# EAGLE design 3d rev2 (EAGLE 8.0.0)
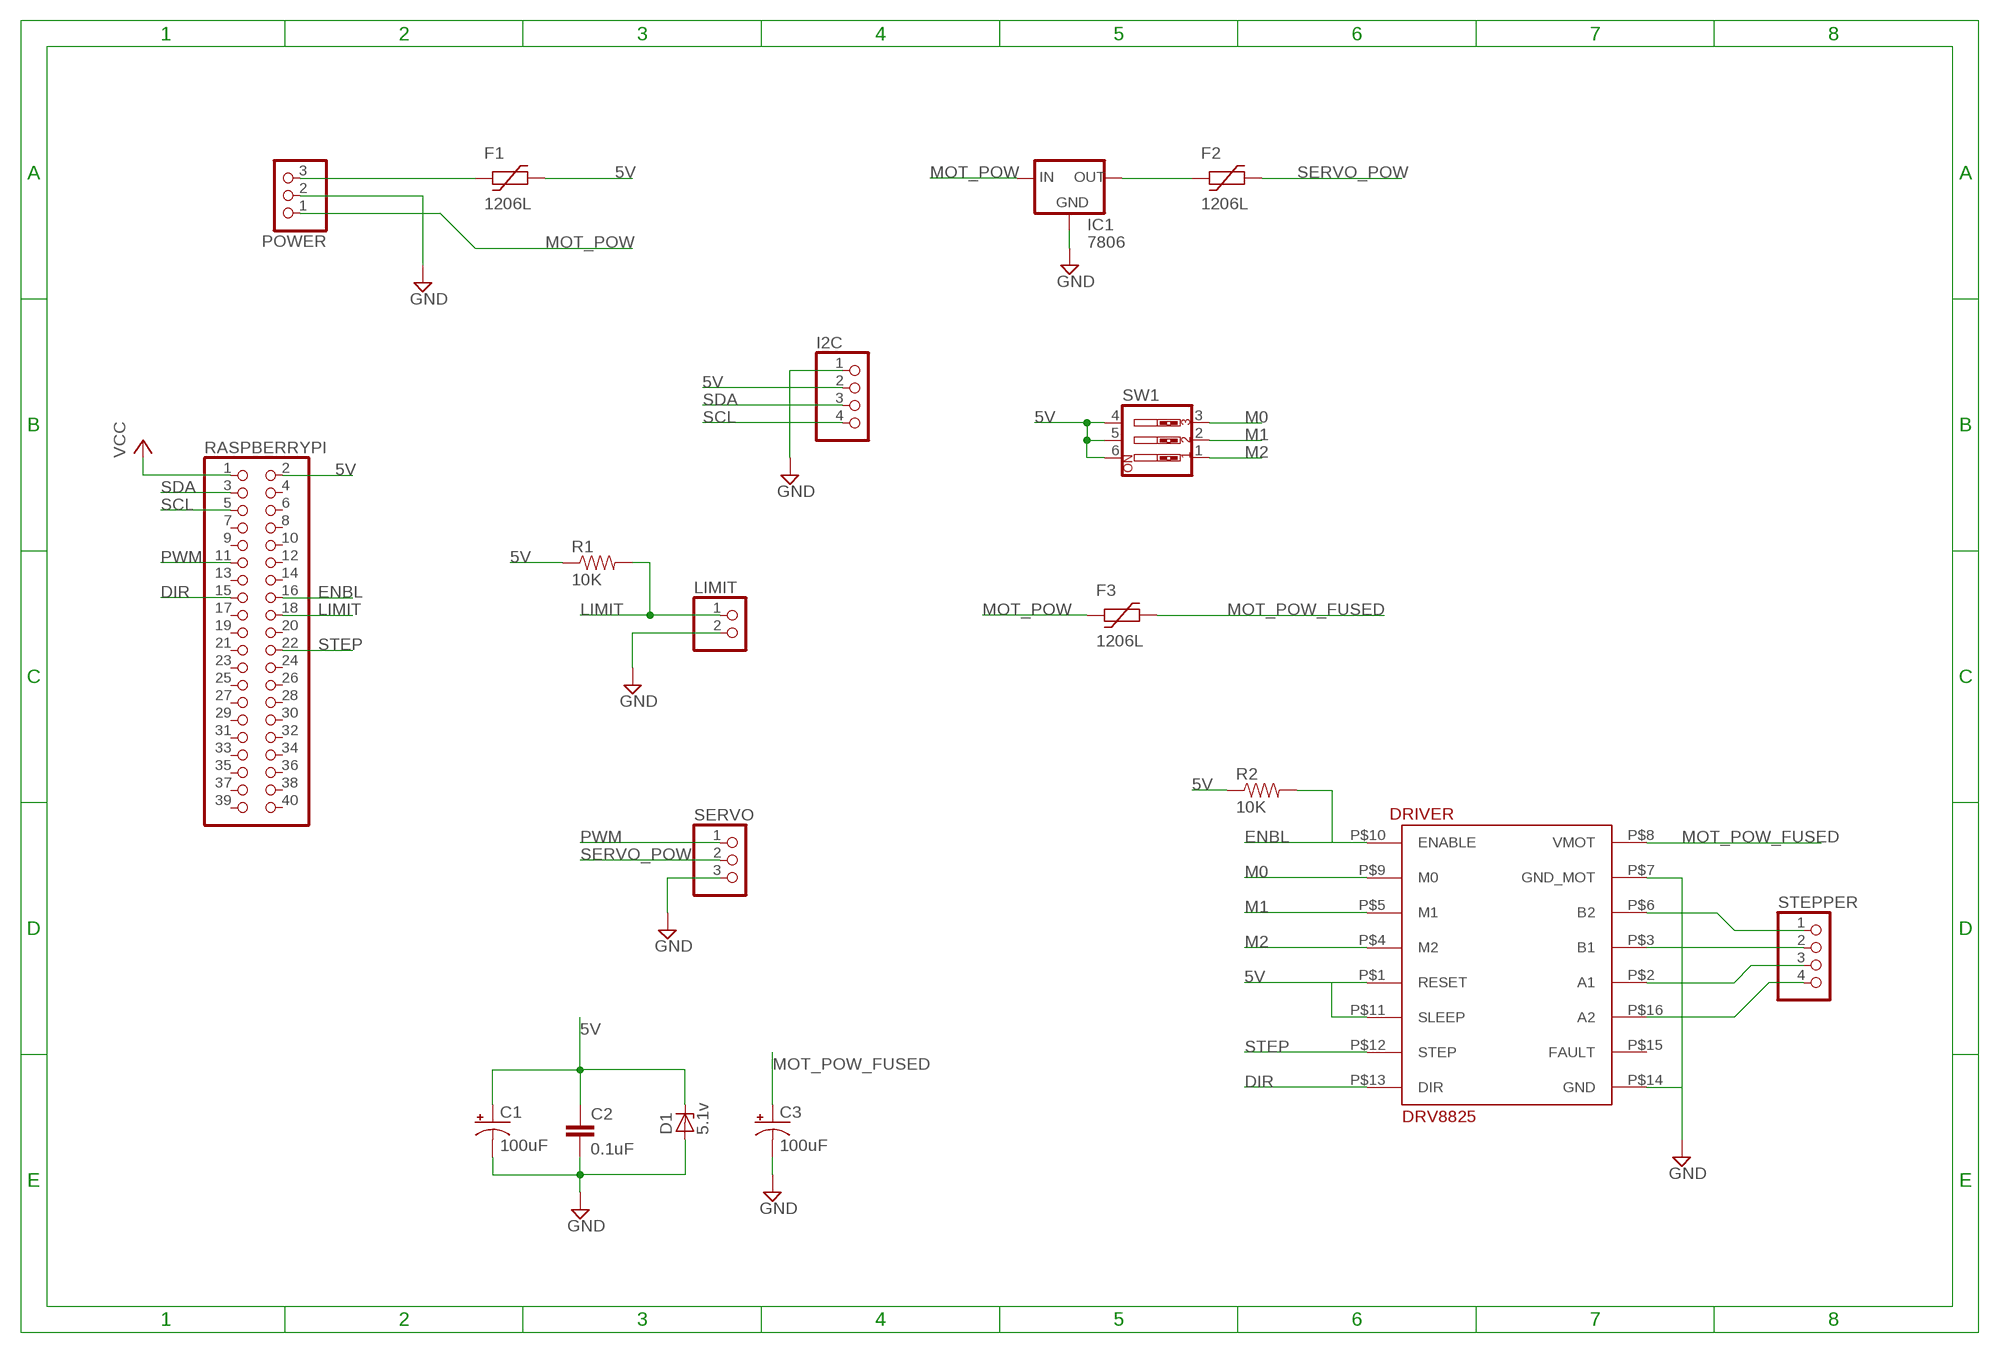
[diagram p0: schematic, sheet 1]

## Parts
C1  100uF  100UF-63V-20%(ELECT)  [NIC_10X10.5_CAP]
C2  0.1uF  0.1UF-25V-5%(0603)  [0603-CAP]
C3  100uF  100UF-63V-20%(ELECT)  [NIC_10X10.5_CAP]
D1  5.1v  ZENER-DIODESOD80C  [SOD80C]
DRIVER  DRV8825  [DRV8825]
F1  1206L  [1206L]
F2  1206L  [1206L]
F3  1206L  [1206L]
I2C  PINHD-1X4  [1X04]
IC1  7806  78LXX  [78LXX]
LIMIT  PINHD-1X2  [1X02]
POWER  PINHD-1X3  [1X03]
R1  10K  RESISTOR1206  [1206]
R2  10K  RESISTOR1206  [1206]
RASPBERRYPI  PINHD-2X20  [2X20]
SERVO  PINHD-1X3  [1X03]
STEPPER  PINHD-1X4  [1X04]
SW1  SW_DIP-3  [EDG-03]

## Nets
5V: C1.+ C2.1 D1.C DRIVER.P$1(RESET) DRIVER.P$11(SLEEP) F1.P$2 I2C.2 R1.1 R2.1 RASPBERRYPI.2 SW1.4 SW1.5 SW1.6
DIR: DRIVER.P$13(DIR) RASPBERRYPI.15
ENBL: DRIVER.P$10(ENABLE) R2.2 RASPBERRYPI.16
GND: C1.- C2.2 C3.- D1.A DRIVER.P$7(GND_MOT) DRIVER.P$14(GND) I2C.1 IC1.GND LIMIT.2 POWER.2 SERVO.3
LIMIT: LIMIT.1 R1.2 RASPBERRYPI.18
M0: DRIVER.P$9(M0) SW1.3
M1: DRIVER.P$5(M1) SW1.2
M2: DRIVER.P$4(M2) SW1.1
MOT_POW: F3.P$1 IC1.IN POWER.1
MOT_POW_FUSED: C3.+ DRIVER.P$8(VMOT) F3.P$2
N$1: DRIVER.P$6(B2) STEPPER.1
N$2: DRIVER.P$3(B1) STEPPER.2
N$3: DRIVER.P$2(A1) STEPPER.3
N$4: DRIVER.P$16(A2) STEPPER.4
N$7: F1.P$1 POWER.3
N$11: F2.P$1 IC1.OUT
PWM: RASPBERRYPI.11 SERVO.1
SCL: I2C.4 RASPBERRYPI.5
SDA: I2C.3 RASPBERRYPI.3
SERVO_POW: F2.P$2 SERVO.2
STEP: DRIVER.P$12(STEP) RASPBERRYPI.22
VCC: RASPBERRYPI.1
Unconnected: DRIVER.P$15(FAULT) RASPBERRYPI.4 RASPBERRYPI.6 RASPBERRYPI.7 RASPBERRYPI.8 RASPBERRYPI.9 RASPBERRYPI.10 RASPBERRYPI.12 RASPBERRYPI.13 RASPBERRYPI.14 RASPBERRYPI.17 RASPBERRYPI.19 RASPBERRYPI.20 RASPBERRYPI.21 RASPBERRYPI.23 RASPBERRYPI.24 RASPBERRYPI.25 RASPBERRYPI.26 RASPBERRYPI.27 RASPBERRYPI.28 RASPBERRYPI.29 RASPBERRYPI.30 RASPBERRYPI.31 RASPBERRYPI.32 RASPBERRYPI.33 RASPBERRYPI.34 RASPBERRYPI.35 RASPBERRYPI.36 RASPBERRYPI.37 RASPBERRYPI.38 RASPBERRYPI.39 RASPBERRYPI.40

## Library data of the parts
C1 C3 = SparkFun-Capacitors:100UF-63V-20%(ELECT): CAP-08362; PROD_ID: CAP-08362
C2 = SparkFun-Capacitors:0.1UF-25V-5%(0603): CAP-08604; PROD_ID: CAP-08604
D1 = diode:ZENER-DIODE: Z-Diode
DRIVER = drv8825 rev2:DRV8825
F1-F3 = ptc-littlefuse:1206L
I2C STEPPER = pinhead:PINHD-1X4: PIN HEADER
IC1 = v-reg:78LXX: VOLTAGE REGULATOR
LIMIT = pinhead:PINHD-1X2: PIN HEADER
POWER SERVO = pinhead:PINHD-1X3: PIN HEADER
R1 R2 = SparkFun-Resistors:RESISTOR: Resistor
RASPBERRYPI = pinhead:PINHD-2X20: PIN HEADER
SW1 = special:SW_DIP-3: DIP SWITCH

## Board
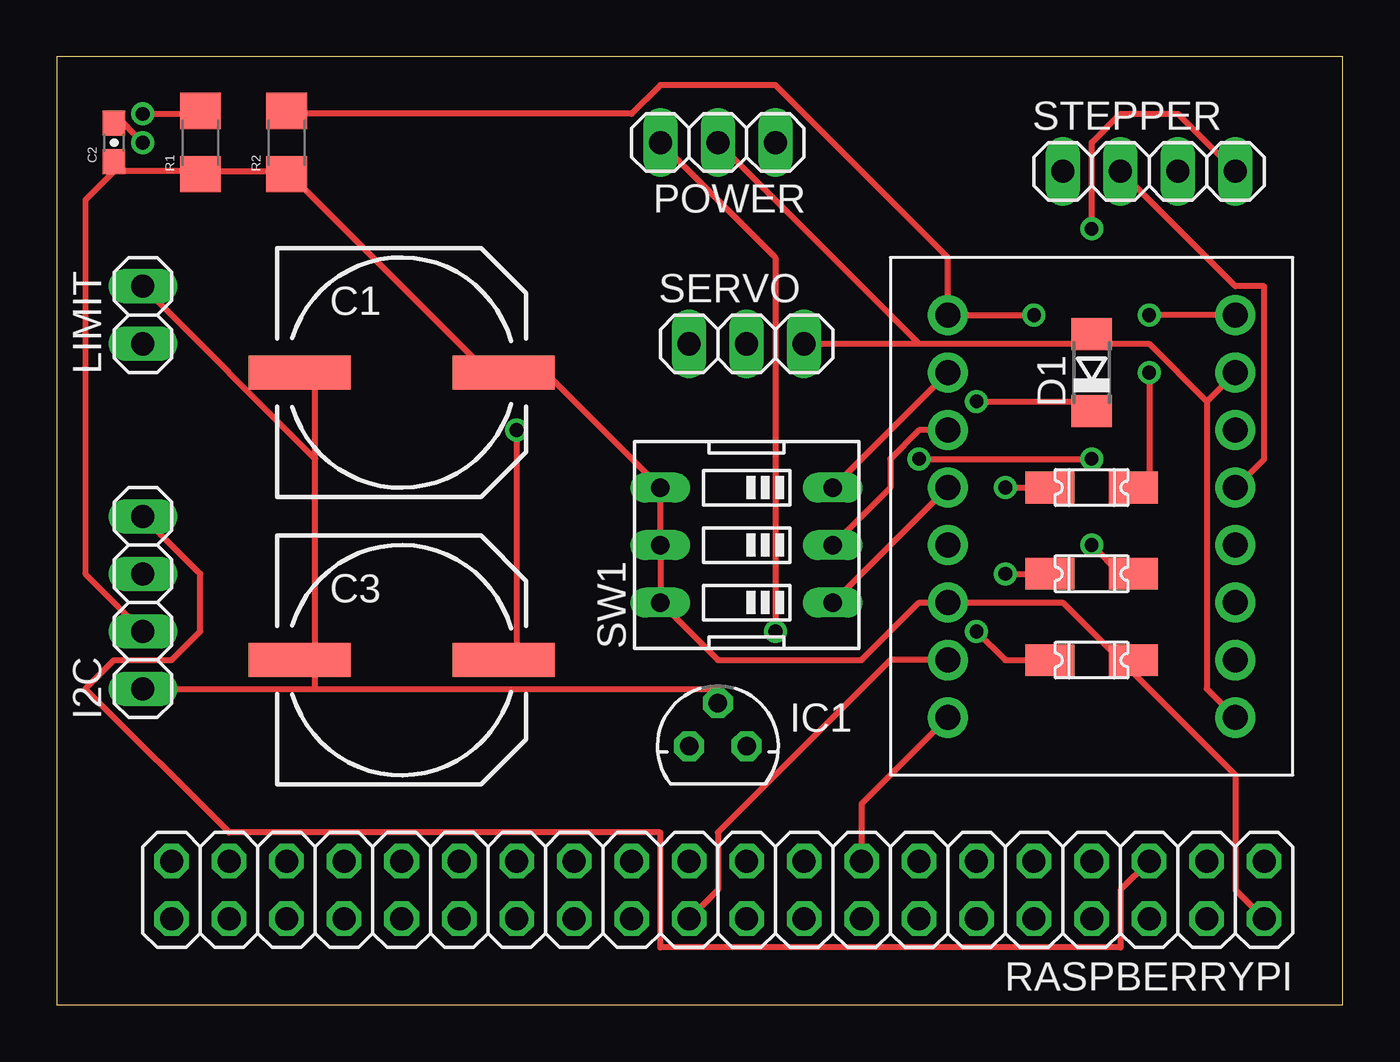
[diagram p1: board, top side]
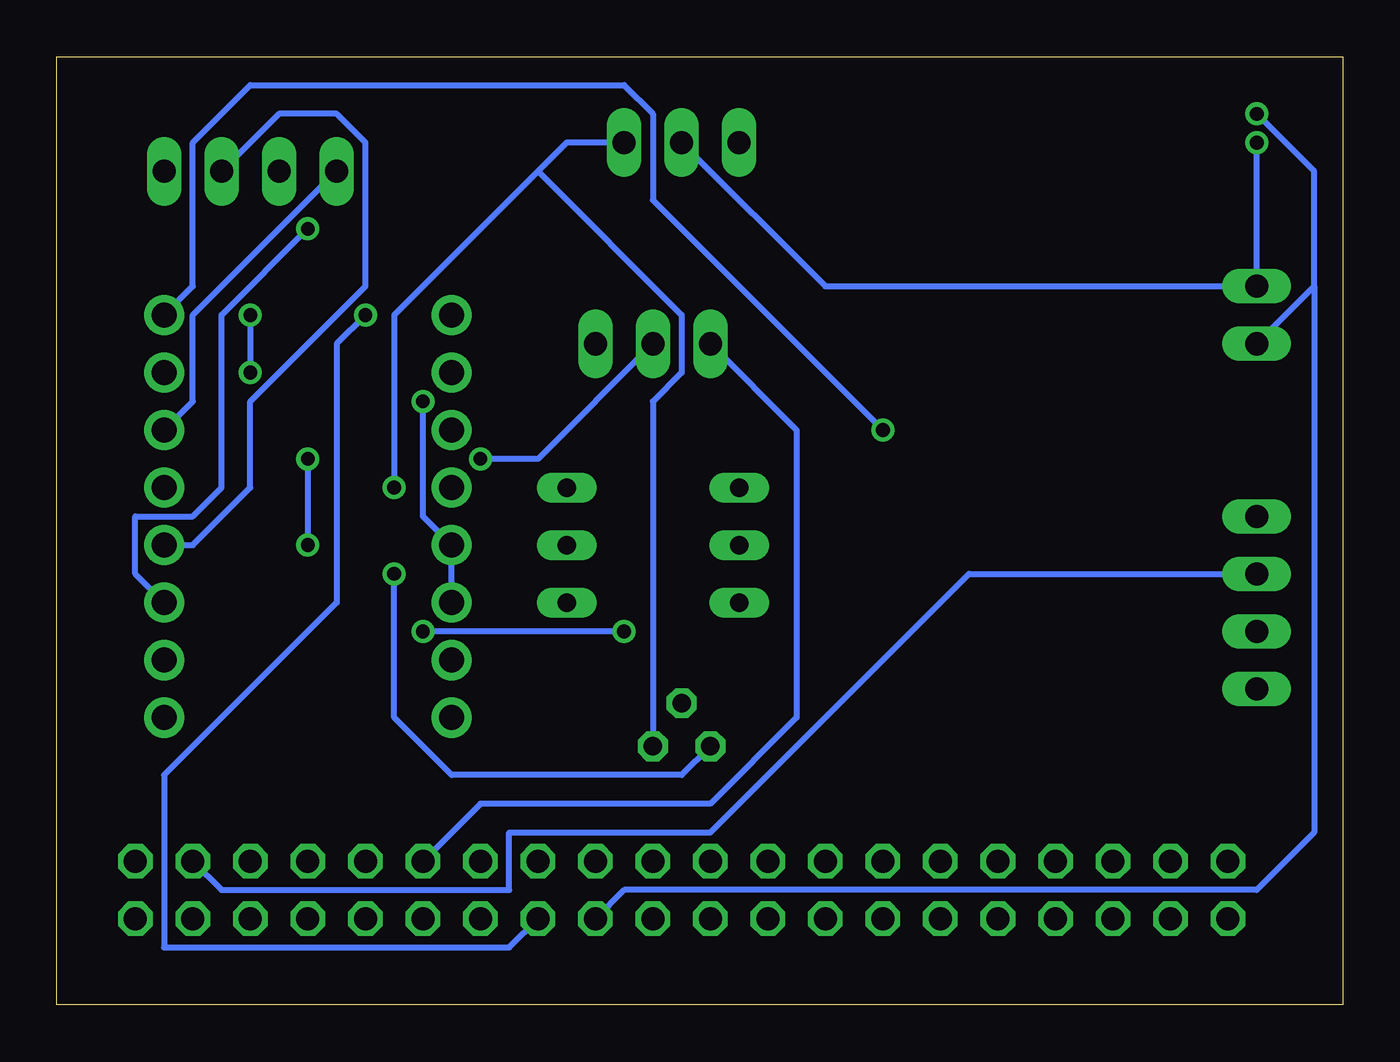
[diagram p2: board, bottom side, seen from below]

Size 56.82 x 41.9 mm. Coordinates in mm from the lower left corner, seen from the top.
Outline: 0,0 56.82,0 56.82,41.9 0,41.9 0,0
Copper layers (1*16): Top 0.035mm / dielectric 1.5mm / Bottom 0.035mm
Design rules "default *": minimum track width 10mil, minimum drill 24mil, track to track 8mil, track to pad 8mil, pad to pad 8mil, via to via 8mil, smd to smd 8mil, copper to edge 40mil, drill to drill 8mil, minimum pad ring 10mil, minimum via ring 8mil, stop-mask expansion 4mil, vias tented up to drill 0mil, thermal gap 10mil

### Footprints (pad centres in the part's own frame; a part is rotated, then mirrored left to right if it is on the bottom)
NIC_10X10.5_CAP = smd 4.5 x 1.5: + 4.5,0; - -4.5,0
0603-CAP = smd 1.1 x 1: 1 -0.85,0; 2 0.85,0
SOD80C = smd 1.4 x 1.8: A 1.7,0; C -1.7,0
DRV8825 = drill 1.1 pad 1.778: P$1 -6.35,-1.27; P$2 6.35,-1.27; P$3 6.35,1.27; P$4 -6.35,1.27; P$5 -6.35,3.81; P$6 6.35,3.81; P$7 6.35,6.35; P$8 6.35,8.89; P$9 -6.35,6.35; P$10 -6.35,8.89; P$11 -6.35,-3.81; P$12 -6.35,-6.35; P$13 -6.35,-8.89; P$14 6.35,-8.89; P$15 6.35,-6.35; P$16 6.35,-3.81
1206L = smd 2.16 x 1.4: P$1 -1.85,0; P$2 1.85,0
1X04 = drill 1.016 long: 1 -3.81,0; 2 -1.27,0; 3 1.27,0; 4 3.81,0
78LXX = drill 0.813 octagon: GND 0,1.905; IN 1.27,0; OUT -1.27,0
1X02 = drill 1.016 long: 1 -1.27,0; 2 1.27,0
1X03 = drill 1.016 long: 1 -2.54,0; 2 0,0; 3 2.54,0
1206 = smd 1.6 x 1.8: 1 -1.4,0; 2 1.4,0
2X20 = drill 1.016 octagon: 1 -24.13,-1.27; 2 -24.13,1.27; 3 -21.59,-1.27; 4 -21.59,1.27; 5 -19.05,-1.27; 6 -19.05,1.27; 7 -16.51,-1.27; 8 -16.51,1.27; 9 -13.97,-1.27; 10 -13.97,1.27; 11 -11.43,-1.27; 12 -11.43,1.27; 13 -8.89,-1.27; 14 -8.89,1.27; 15 -6.35,-1.27; 16 -6.35,1.27; 17 -3.81,-1.27; 18 -3.81,1.27; 19 -1.27,-1.27; 20 -1.27,1.27; 21 1.27,-1.27; 22 1.27,1.27; 23 3.81,-1.27; 24 3.81,1.27; 25 6.35,-1.27; 26 6.35,1.27; 27 8.89,-1.27; 28 8.89,1.27; 29 11.43,-1.27; 30 11.43,1.27; 31 13.97,-1.27; 32 13.97,1.27; 33 16.51,-1.27; 34 16.51,1.27; 35 19.05,-1.27; 36 19.05,1.27; 37 21.59,-1.27; 38 21.59,1.27; 39 24.13,-1.27; 40 24.13,1.27
EDG-03 = drill 0.813 long: 1 -2.54,-3.81; 2 0,-3.81; 3 2.54,-3.81; 4 2.54,3.81; 5 0,3.81; 6 -2.54,3.81

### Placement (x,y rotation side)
C1  15.24,27.94 0 top
C2  2.54,38.1 90 top
C3  15.24,15.24 0 top
D1  45.72,27.94 90 top
DRIVER  45.72,21.59 0 top
F1  45.72,15.24 0 top
F2  45.72,19.05 0 top
F3  45.72,22.86 0 top
I2C  3.81,17.78 90 top
IC1  29.21,11.43 0 top
LIMIT  3.81,30.48 90 top
POWER  29.21,38.1 180 top
R1  6.35,38.1 90 top
R2  10.16,38.1 90 top
RASPBERRYPI  29.21,5.08 180 top
SERVO  30.48,29.21 0 top
STEPPER  48.26,36.83 0 top
SW1  30.48,20.32 90 top

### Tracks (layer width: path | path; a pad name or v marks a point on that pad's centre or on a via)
5V  (via drill 0.61)
  Top 0.254: v40.64,26.67 45.72,26.67 D1.C | 46.99,15.24 44.45,17.78 DRIVER.P$11 38.1,17.78 35.56,15.24 29.21,15.24 SW1.6 SW1.5 SW1.4 21.59,27.94 C1.+ 19.05,27.94 10.16,36.83 | RASPBERRYPI.2 52.07,5.08 52.07,10.16 46.99,15.24 | 46.99,15.24 F1.P$2 | 6.35,36.83 2.54,36.83 | 6.35,36.83 10.16,36.83 | 6.35,36.83 R1.1 | I2C.2 1.27,19.05 1.27,35.56 2.54,36.83 | 2.54,36.83 C2.1 | 10.16,36.83 R2.1
  Bottom 0.254: v40.64,26.67 40.64,21.59 DRIVER.P$1 DRIVER.P$11
DIR
  Top 0.254: RASPBERRYPI.15 35.56,8.89 DRIVER.P$13
ENBL  (via drill 0.61)
  Top 0.254: R2.2 10.16,39.37 25.4,39.37 26.67,40.64 31.75,40.64 39.37,33.02 DRIVER.P$10 v43.18,30.48
  Bottom 0.254: RASPBERRYPI.16 36.83,2.54 52.07,2.54 52.07,10.16 44.45,17.78 44.45,29.21 v43.18,30.48
GND  (via drill 0.61)
  Top 0.254: v3.81,38.1 2.54,39.37 C2.2 | I2C.1 11.43,13.97 | 11.43,13.97 29.21,13.97 IC1.GND | 11.43,13.97 11.43,15.24 | 11.43,15.24 11.43,24.13 | 11.43,24.13 11.43,27.94 C1.- | 11.43,15.24 C3.- | 11.43,24.13 LIMIT.2 | DRIVER.P$14 50.8,13.97 50.8,26.67 | DRIVER.P$7 50.8,26.67 | SERVO.3 38.1,29.21 | 38.1,29.21 45.72,29.21 | 38.1,29.21 POWER.2 | 50.8,26.67 48.26,29.21 45.72,29.21 | 45.72,29.21 D1.A
  Bottom 0.254: v3.81,38.1 LIMIT.2 22.86,31.75 POWER.2
LIMIT  (via drill 0.61)
  Top 0.254: v3.81,39.37 6.35,39.37 R1.2
  Bottom 0.254: v3.81,39.37 1.27,36.83 1.27,31.75 | LIMIT.1 1.27,31.75 | RASPBERRYPI.18 31.75,5.08 3.81,5.08 1.27,7.62 1.27,31.75
M0
  Top 0.254: DRIVER.P$9 SW1.3
M1
  Top 0.254: SW1.2 36.83,22.86 36.83,24.13 38.1,25.4 DRIVER.P$5
M2
  Top 0.254: DRIVER.P$4 SW1.1
MOT_POW  (via drill 0.61)
  Top 0.254: v41.91,22.86 F3.P$1
  Bottom 0.254: v41.91,22.86 41.91,30.48 35.56,36.83 | 35.56,36.83 34.29,38.1 POWER.1 | IC1.IN 30.48,26.67 29.21,27.94 29.21,30.48 35.56,36.83
MOT_POW_FUSED  (via drill 0.61)
  Top 0.254: v48.26,27.94 48.26,22.86 F3.P$2 | DRIVER.P$8 v48.26,30.48 | v20.32,25.4 20.32,15.24 C3.+
  Bottom 0.254: v48.26,30.48 v48.26,27.94 | v20.32,25.4 30.48,35.56 30.48,39.37 31.75,40.64 48.26,40.64 50.8,38.1 50.8,31.75 DRIVER.P$8
N$1
  Bottom 0.254: STEPPER.1 50.8,30.48 50.8,26.67 DRIVER.P$6
N$2
  Top 0.254: STEPPER.2 52.07,31.75 53.34,31.75 53.34,24.13 DRIVER.P$3
N$3
  Bottom 0.254: STEPPER.3 46.99,39.37 44.45,39.37 43.18,38.1 43.18,31.75 48.26,26.67 48.26,22.86 50.8,20.32 DRIVER.P$2
N$4  (via drill 0.61)
  Top 0.254: STEPPER.4 49.53,39.37 46.99,39.37 45.72,38.1 v45.72,34.29
  Bottom 0.254: v45.72,34.29 49.53,30.48 49.53,22.86 50.8,21.59 53.34,21.59 53.34,19.05 DRIVER.P$16
N$7  (via drill 0.61)
  Top 0.254: F1.P$1 41.91,15.24 v40.64,16.51 | v31.75,16.51 31.75,33.02 POWER.3
  Bottom 0.254: v31.75,16.51 v40.64,16.51
N$11  (via drill 0.61)
  Top 0.254: v41.91,19.05 F2.P$1
  Bottom 0.254: v41.91,19.05 41.91,12.7 39.37,10.16 29.21,10.16 IC1.OUT
PWM
  Bottom 0.254: RASPBERRYPI.11 38.1,8.89 27.94,8.89 24.13,12.7 24.13,25.4 SERVO.1
SCL
  Top 0.254: I2C.4 6.35,19.05 6.35,16.51 5.08,15.24 2.54,15.24 1.27,13.97 7.62,7.62 26.67,7.62 26.67,2.54 46.99,2.54 46.99,5.08 RASPBERRYPI.5
SDA
  Bottom 0.254: I2C.3 16.51,19.05 27.94,7.62 36.83,7.62 36.83,5.08 49.53,5.08 RASPBERRYPI.3
SERVO_POW  (via drill 0.61)
  Top 0.254: v45.72,20.32 46.99,19.05 F2.P$2 | v38.1,24.13 v45.72,24.13
  Bottom 0.254: v45.72,24.13 v45.72,20.32 | v38.1,24.13 35.56,24.13 SERVO.2
STEP
  Top 0.254: RASPBERRYPI.22 29.21,5.08 29.21,7.62 36.83,15.24 DRIVER.P$12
